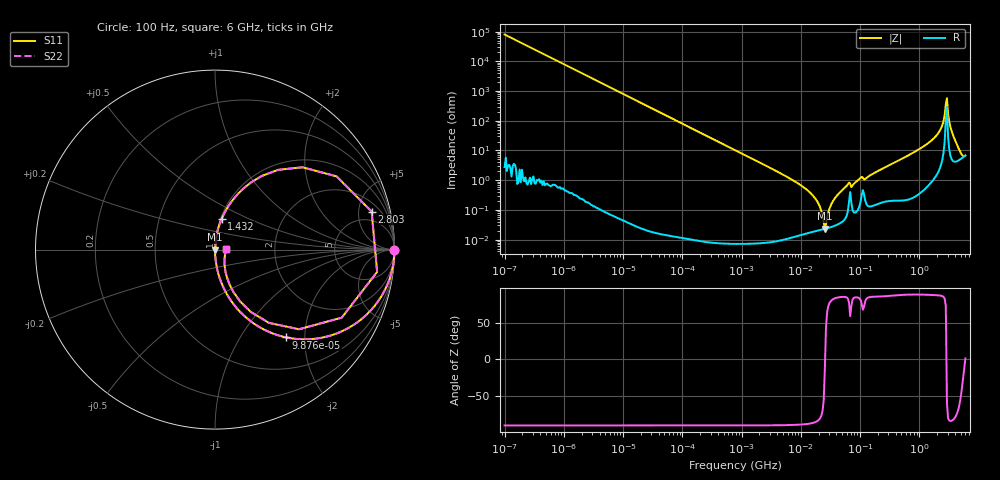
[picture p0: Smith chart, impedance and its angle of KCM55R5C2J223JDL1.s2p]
!Murata Part Number: KCM55R5C2J223JDL1
!These Parameters are Measured in Series Mode Connection
!Data Generated on Mar 13, 2026
!  o--ll--o
!Port1  Port2
!  o------o
!Operation Temp=25[degC], DC Bias Voltage=0[V]
!Freq. Start=100[Hz] Stop=6[GHz] 401[Steps]
# Hz S RI R 50
!Freq.(Hz) S11(Real) S11(Imag) S21(Real) S21(Imag) S12(Real) S12(Imag) S22(Real) S22(Imag)
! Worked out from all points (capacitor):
!   401 points, 100 Hz to 6 GHz, reference 50 ohm
!   read as one part in series: C = 19.9 nF near 109 Hz
!   lowest |Z| = 23.5 mohm at 25.46 MHz (marker M1)
!   series resonance near 25.67 MHz, so ESL is about 1.9 nH
!   S11 on the Smith chart (normalised r, x): 100 Hz: open; 98.76 kHz: 1.00, -1.62; 1.432 GHz: 1.01, +0.36; 2.803 GHz: 3.17, +6.94; 6 GHz: 1.14, +0.00
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100  1 -0.00125  1.6e-06 0.00125  1.6e-06 0.00125  1 -0.00125
2008  0.9994 -0.025  0.000629 0.025  0.000629 0.025  0.9994 -0.025
40335  0.7979 -0.4015  0.2021 0.4015  0.2021 0.4015  0.7979 -0.4015
98762  0.3972 -0.4892  0.6028 0.4892  0.6028 0.4892  0.3972 -0.4892
231233  0.1073 -0.3094  0.8927 0.3094  0.8927 0.3094  0.1073 -0.3094
774597  0.0106 -0.1023  0.9894 0.1023  0.9894 0.1023  0.0106 -0.1023
6644369  0.000239 -0.0112  0.9998 0.0112  0.9998 0.0112  0.000239 -0.0112
1.555665e7  0.000191 -0.00323  0.9998 0.00323  0.9998 0.00323  0.000191 -0.00323
2.035112e7  0.000207 -0.00145  0.9998 0.00145  0.9998 0.00145  0.000207 -0.00145
2.545746e7  0.000229 -5.15e-05  0.9998 5.15e-05  0.9998 5.15e-05  0.000229 -5.15e-05
3.482834e7  0.000281 0.00193  0.9997 -0.00193  0.9997 -0.00193  0.000281 0.00193
5.960426e7  0.000688 0.00646  0.9993 -0.00646  0.9993 -0.00646  0.000688 0.00646
3.124326e8  0.00299 0.0316  0.997 -0.0316  0.997 -0.0316  0.00299 0.0316
1.431855e9  0.0375 0.1724  0.9625 -0.1724  0.9625 -0.1724  0.0375 0.1724
2.048624e9  0.1281 0.311  0.8719 -0.311  0.8719 -0.311  0.1281 0.311
2.450438e9  0.3516 0.4443  0.6484 -0.4443  0.6484 -0.4443  0.3516 0.4443
2.802721e9  0.8727 0.2119  0.1273 -0.2119  0.1273 -0.2119  0.8727 0.2119
3.065283e9  0.7062 -0.379  0.2938 0.379  0.2938 0.379  0.7062 -0.379
3.352442e9  0.3005 -0.4082  0.6995 0.4082  0.6995 0.4082  0.3005 -0.4082
4.009986e9  0.0806 -0.1931  0.9194 0.1931  0.9194 0.1931  0.0806 -0.1931
5.016141e9  0.0528 -0.0578  0.9472 0.0578  0.9472 0.0578  0.0528 -0.0578
6e9  0.0633 0.00124  0.9367 -0.00124  0.9367 -0.00124  0.0633 0.00124
